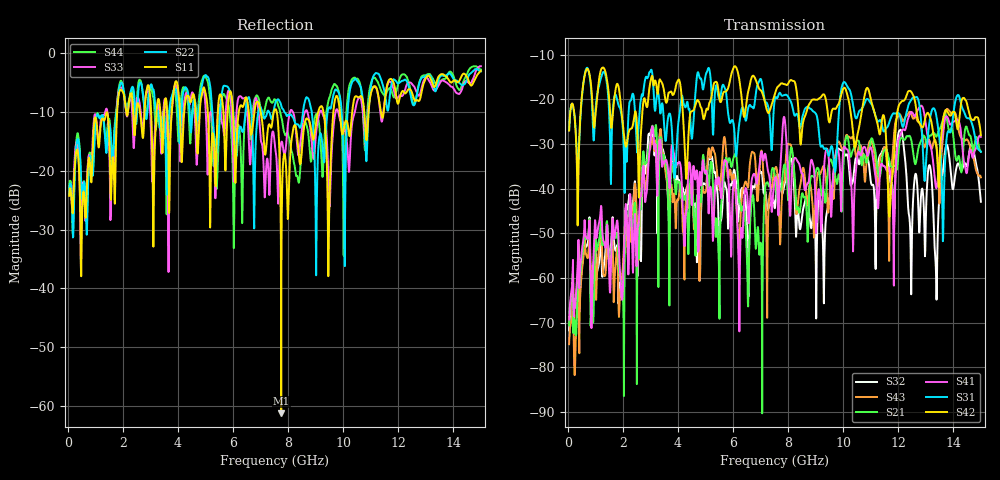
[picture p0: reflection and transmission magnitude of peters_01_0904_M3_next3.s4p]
# MHZ S RI R 50.00
! FREQ  S11  S12  S13  S14
!  S21  S22  S23  S24
!  S31  S32  S33  S34
!  S41  S42  S43  S44
!  REAL  IMAG  REAL  IMAG  REAL  IMAG  REAL  IMAG
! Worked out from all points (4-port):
!   1496 points, 50 MHz to 15 GHz, reference 50 ohm
!   strongest paths, dB at 50 MHz, 3.79 GHz, 7.53 GHz, 11.27 GHz, 15 GHz:
!     S42: -27.0, -18.7, -18.6, -26.1, -28.0
!     S31: -26.9, -27.9, -19.7, -25.0, -31.7
!     S41: -69.3, -30.2, -37.6, -44.4, -28.4
!     S21: -70.6, -35.0, -37.5, -36.5, -31.7
!     S43: -74.8, -40.8, -35.4, -38.2, -37.5
!     S32: -71.7, -32.9, -44.1, -34.4, -42.9
!   lowest |S11| = -61.2 dB at 7.75 GHz (marker M1), VSWR 1.00, Z = 49.9 - j0.0453 ohm
!   |S11| at or under -10 dB: start of sweep to 1.794 GHz; 7.002 GHz to 7.484 GHz (482.1 MHz wide, 6.66 % of centre); 7.587 GHz to 9.096 GHz (1.509 GHz wide, 18.1 % of centre)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
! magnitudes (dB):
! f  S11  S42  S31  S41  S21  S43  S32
! 50 MHz  -24.3  -27.0  -26.9  -69.3  -70.6  -74.8  -71.7
! 1.99 GHz  -6.5  -25.0  -25.7  -63.9  -63.8  -58.4  -62.8
! 3.06 GHz  -14.9  -14.7  -13.8  -26.2  -26.1  -28.6  -27.1
! 6.24 GHz  -9.3  -16.0  -24.9  -63.6  -43.0  -52.1  -42.7
! 7.75 GHz  -61.2  -16.4  -19.0  -32.4  -40.1  -45.4  -40.1
! 11.69 GHz  -4.5  -45.6  -24.8  -35.8  -34.1  -44.5  -37.2
! 15 GHz  -3.1  -28.0  -31.7  -28.4  -31.7  -37.5  -42.9
